ORGANIZATION_BLOCK "CYCL_EXC"
TITLE = "Main Program Sweep (Cycle)"
//Abstract:
//Example for data transmission to Siebert C9030 Profibus-DP Gagteway.
//
//This example shows how to transmit data to two gateways.
//Assign one DB of 76 bytes length to each gateway for data transmission (SendDb)
//(in this example DB1 and DB2).
//Data must be stored in DB's containing only one string (DB3, DB4, DB5).
//
//Call function "Send_Data" every cycle with number of SendDb for each gateway.
//Function "Send_Data" handles handshake, segmentation and transmission of data.
//Function  returns 0 when transmission is completed and new data can be sent,
//error code else (see function description).
//
//Call function "Set_Tx_Data" to set new data. Function "Set_Tx_Data" stores info
//for data transmission in the SendDb for one gateway and initiates transmission
//of data to that gateway.
VERSION : 0.1


VAR_TEMP
  OB1_EV_CLASS : BYTE ;	//Bits 0-3 = 1 (Coming event), Bits 4-7 = 1 (Event class 1)
  OB1_SCAN_1 : BYTE ;	//1 (Cold restart scan 1 of OB 1), 3 (Scan 2-n of OB 1)
  OB1_PRIORITY : BYTE ;	//Priority of OB Execution
  OB1_OB_NUMBR : BYTE ;	//1 (Organization block 1, OB1)
  OB1_RESERVED_1 : BYTE ;	//Reserved for system
  OB1_RESERVED_2 : BYTE ;	//Reserved for system
  OB1_PREV_CYCLE : INT ;	//Cycle time of previous OB1 scan (milliseconds)
  OB1_MIN_CYCLE : INT ;	//Minimum cycle time of OB1 (milliseconds)
  OB1_MAX_CYCLE : INT ;	//Maximum cycle time of OB1 (milliseconds)
  OB1_DATE_TIME : DATE_AND_TIME ;	//Date and time OB1 started
  T_OutputAddr1 : WORD ;	//Temp storage for configured output data area
  T_InputAddr1 : WORD ;	//Temp storage for configured input data area
  T_SendDb1 : INT ;	//Temp storage for number of SendDb
  T_OutputLen1 : INT ;	//Temp storage for configured length of output data
  T_OutputAddr2 : WORD ;	//Temp storage for configured output data area
  T_InputAddr2 : WORD ;	//Temp storage for configured input data area
  T_SendDb2 : INT ;	//Temp storage for number of SendDb
  T_OutputLen2 : INT ;	//Temp storage for configured length of output data
  T_SourceDb : INT ;	//Temp storage for number of SourceDb
END_VAR
BEGIN
NETWORK
TITLE =Set configuration dependent variables
//Set temporary variables for data exchange with gateway to fixed values
//according to hardware configuration.
//
//These settings must be changed to match the hardware configuration.
//Settings for this example are:
//
//Gateway 1:     Output Address Start  40 (28hex)
//               Input Address         2
//               SendDb                SendDb1 (DB1)
//               Ouput Data Length     2 (Online Text 1 In 2 Out con)
//
//Gateway 2:     Output Address Start  80 (50hex)
//               Input Address         3
//               SendDb                SendDb2 (DB2)
//               Ouput Data Length     8 (Online Text 1 In 8 Out con)

// ** set values for gateway 1
      L     W#16#28; // load output data area start address as set in hardware configuration
      T     #T_OutputAddr1; // store tmp

      L     W#16#2; // load input data area start address as set in hardware configuration
      T     #T_InputAddr1; // store tmp

      L     W#16#1; // load number of Send Db
      T     #T_SendDb1; // store tmp

      L     W#16#2; // load output data length as set in hardware configuration
      T     #T_OutputLen1; // store tmp

// ** set values for gateway 2
      L     W#16#50; // load output data area start address as set in hardware configuration
      T     #T_OutputAddr2; // store tmp

      L     W#16#3; // load input data area start address as set in hardware configuration
      T     #T_InputAddr2; // store tmp

      L     W#16#2; // load number of Send Db
      T     #T_SendDb2; // store tmp

      L     W#16#8; // load output data length as set in hardware configuration
      T     #T_OutputLen2; // store tmp

NETWORK
TITLE =Handling and data transmission to gateway 1
//Call function Send_Data to transmit data to gateway, data is transmitted
//consistently. Function is called with the number of the SendDb for one gateway.
//Return value is 0 when new data can be sent (i.e. former transmission is
//completed).
//
//Call function "Set_Tx_Data" to initiate transmission of new data. Function is
//called with the following variables
//
//OutputAddr:  first address of gateway outputs
//InputAddr:   address of gateway input
//SrcDb:       number of source DB (contains data string to be sent)
//SendDb:      number of send DB for gateway
//LenConsData: lenght of consistent data, MUST EQUAL LENGTH FOR CONFIGURED MODULE
//RETVAL:      return value from function; 0 if ok, error else
//             (see description in function)

// ** call function "Send_Data" for transmission of data to gateway
// ** return value signals if transmission is completed and new data can be sent

      CALL "Send_Data" (// call function every cycle to proceed data transmission
           SendDb                   := #T_SendDb1,// SendDb contains information about data to send
           RETVAL                   := MW   200);// function returns 0 if transmission completed

      L     MW   200; // load return value
      L     W#16#0; // load compare value
      <>I   ; // return value unequal 0 ?
      SPB   L299; // jump if busy condition or any error reported

// ** check inputs to set transmission data on input event
      U     E      0.0;
      FP    M    199.0; // positive edge on input ?
      SPBN  L201; // no --> check next input
      L     W#16#3; // load number of DB containing data to send (source DB)
      T     MW   190; // store number of source DB
      SPA   L290; // send data

L201: U     E      0.1;
      FP    M    199.1; // positive edge on input ?
      SPBN  L202; // no --> check next input
      L     W#16#4; // load number of DB containing data to send (source DB)
      T     MW   190; // store number of source DB
      SPA   L290; // send data

L202: U     E      0.2;
      FP    M    199.2; // positive edge on input ?
      SPBN  L299; // no --> jump out
      L     W#16#5; // load number of DB containing data to send (source DB)
      T     MW   190; // store number of source DB
      SPA   L290; // send data

// ** call function "Set_Tx_Data" to initiate transmission of data to gateway
L290: NOP   0;

      L     MW   190; // get number of DB set from inputs
      T     #T_SourceDb; // store tmp

      CALL "Set_Tx_Data" (
           OutputAddr               := #T_OutputAddr1,
           InputAddr                := #T_InputAddr1,
           SrcDb                    := #T_SourceDb,
           SendDb                   := #T_SendDb1,
           LenConsData              := #T_OutputLen1,
           RETVAL                   := MW   200);

// ** check return value for errors (see function description of error codes)
// ** insert additional treatment for errors if necessary

      L     MW   200; // load return value
      L     W#16#0; // load compare value
      ==I   ; // return value 0x0000 ?
      SPB   ERR1;
      SPA   L299; // jump out

L299: NOP   0;
      SPA   NW3; // goto next network

ERR1: NOP   0;
      SPA   NW3; // goto next network (no error handling)

NETWORK
TITLE =Handling and data transmission to gateway 2
//Call function Send_Data to transmit data to gateway, data is transmitted
//consistently. Function is called with the number of the SendDb for one gateway.
//Return value is 0 when new data can be sent (i.e. former transmission is
//completed).
//
//Call function "Set_Tx_Data" to initiate transmission of new data. Function is
//called with the following variables
//
//OutputAddr:  first address of gateway outputs
//InputAddr:   address of display input
//SrcDb:       number of source DB (contains data string to be sent)
//SendDb:      number of send DB for gateway
//LenConsData: lenght of consistent data, MUST EQUAL LENGTH FOR CONFIGURED MODULE
//RETVAL:      return value from function; 0 if ok, error else
//             (see description in function)
NW3:  NOP   0;

// ** call function "Send_Data" for transmission of data to gateway
// ** return value signals if transmission is completed and new data can be sent

      CALL "Send_Data" (// call function every cycle to proceed data transmission
           SendDb                   := #T_SendDb2,// SendDb contains information about data to send
           RETVAL                   := MW   202);// function returns 0 if transmission completed

      L     MW   202;
      L     W#16#0;
      <>I   ;
      SPB   L399; // jump if any error reported

// ** check inputs to set transmission data on input event
      U     E      0.3;
      FP    M    199.3; // positive edge on input ?
      SPBN  L301; // no --> check next input
      L     W#16#3; // load number of DB containing data to send (source DB)
      T     MW   190; // store number of source DB
      SPA   L390; // send data

L301: U     E      0.4;
      FP    M    199.4; // positive edge on input ?
      SPBN  L302; // no --> check next input
      L     W#16#4; // load number of DB containing data to send (source DB)
      T     MW   190; // store number of source DB
      SPA   L390; // send data

L302: U     E      0.5;
      FP    M    199.5; // positive edge on input ?
      SPBN  L399; // no --> jump out
      L     W#16#5; // load number of DB containing data to send (source DB)
      T     MW   190; // store number of source DB
      SPA   L390; // send data

// ** call function "Set_Tx_Data" to initiate transmission of data to gateway
L390: NOP   0;

      L     MW   190; // get number of DB set from inputs
      T     #T_SourceDb; // store tmp

      CALL "Set_Tx_Data" (
           OutputAddr               := #T_OutputAddr2,
           InputAddr                := #T_InputAddr2,
           SrcDb                    := #T_SourceDb,
           SendDb                   := #T_SendDb2,
           LenConsData              := #T_OutputLen2,
           RETVAL                   := MW   202);

// ** check return value for errors (see function description of error codes)
// ** insert additional treatment for errors if necessary

      L     MW   202; // load return value
      L     W#16#0; // load compare value
      ==I   ; // return value 0x0000 ?
      SPB   ERR2;
      SPA   L399; // jump out

L399: NOP   0;
      BE    ; // quit

ERR2: NOP   0;
      BE    ; // no error handling

END_ORGANIZATION_BLOCK

